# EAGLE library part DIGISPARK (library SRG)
Digispark http://digistump.com/wiki/digispark
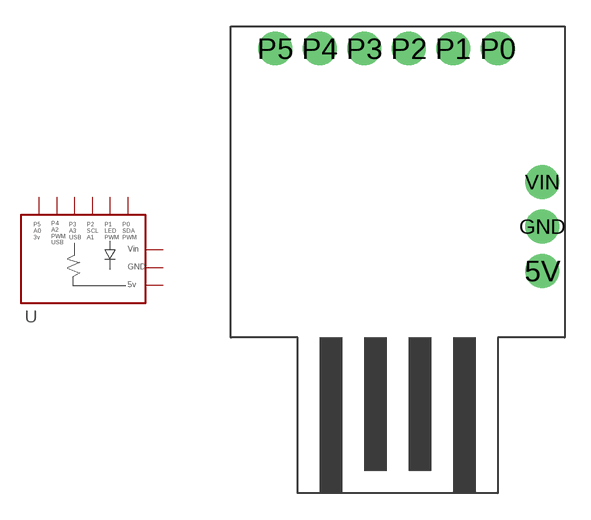
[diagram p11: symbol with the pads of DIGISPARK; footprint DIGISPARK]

Designator prefix -

## DIGISPARK  [DIGISPARK]
5V  5V  pwr
GND  GND  pwr
P0  P0
P1  P1
P2  P2
P3  P3
P4  P4
P5  P5
VIN  VIN  pwr

## Footprint DIGISPARK (pad centres in mm)
DigiSpark
drill 1 pad 1.93: 5V 17.78,3.81; GND 17.78,6.35; P0 15.24,16.51; P1 12.7,16.51; P2 10.16,16.51; P3 7.62,16.51; P4 5.08,16.51; P5 2.54,16.51; VIN 17.78,8.89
